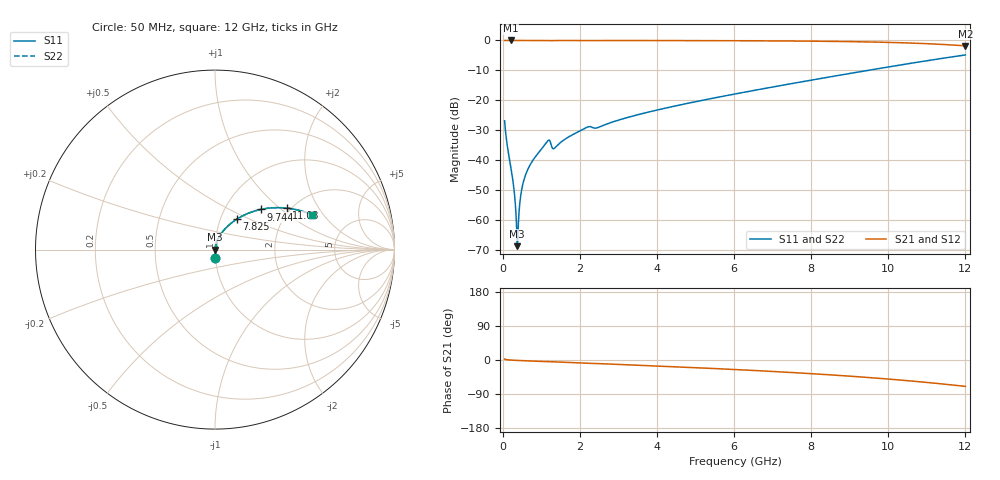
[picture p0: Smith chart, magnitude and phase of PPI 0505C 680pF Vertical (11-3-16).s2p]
# GHz S MA R 50
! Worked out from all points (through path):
!   1601 points, 50 MHz to 12 GHz, reference 50 ohm
!   highest |S21| = 0.00 dB at 214.3 MHz (marker M1); lowest = -1.8 dB at 12 GHz (marker M2)
!   group delay of S21, straight-line fit = 15.2 ps
!   lowest |S11| = -68.6 dB at 378.6 MHz (marker M3), VSWR 1.00, Z = 50 - j0.00888 ohm
!   |S11| at or under -10 dB: start of sweep to 9.462 GHz
!   |S22| runs from -68.6 to -4.8 dB; largest |S21 - S12| = 0
!   S11 on the Smith chart (normalised r, x): 50 MHz: 1.00, -0.09; 7.825 GHz: 1.19, +0.42; 9.744 GHz: 1.46, +0.74; 11.03 GHz: 1.90, +1.12; 12 GHz: 2.68, +1.56
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0.05  0.04591 -87.3  0.9987 2.5  0.9987 2.5  0.04591 -87.3
0.2143125  0.007481 -87.9  0.9997 -0.2  0.9997 -0.2  0.007481 -87.9
0.2815313  0.003802 -85.7  0.9996 -0.6  0.9996 -0.6  0.003802 -85.7
0.3412812  0.00141 -76.6  0.9996 -0.9  0.9996 -0.9  0.00141 -76.6
0.378625  0.0003727 -13.8  0.9996 -1.1  0.9996 -1.1  0.0003727 -13.8
0.4159687  0.001147 69.5  0.9996 -1.3  0.9996 -1.3  0.001147 69.5
0.4831875  0.003002 80.7  0.9996 -1.6  0.9996 -1.6  0.003002 80.7
0.5504062  0.004708 82.9  0.9995 -1.9  0.9995 -1.9  0.004708 82.9
0.6624375  0.00734 84.0  0.9995 -2.4  0.9995 -2.4  0.00734 84.0
0.8192812  0.01086 84.0  0.9993 -3.1  0.9993 -3.1  0.01086 84.0
1.162844  0.02094 74.3  0.9957 -4.6  0.9957 -4.6  0.02094 74.3
1.342094  0.01596 71.5  0.996 -4.9  0.996 -4.9  0.01596 71.5
2.044156  0.03209 79.1  0.9977 -7.9  0.9977 -7.9  0.03209 79.1
2.454938  0.03506 74.4  0.9954 -9.3  0.9954 -9.3  0.03506 74.4
4.038312  0.07005 73.0  0.996 -16.0  0.996 -16.0  0.07005 73.0
6.025  0.1282 64.2  0.9898 -25.1  0.9898 -25.1  0.1282 64.2
7.824969  0.2082 54.5  0.9755 -35.0  0.9755 -35.0  0.2082 54.5
8.019156  0.219 53.3  0.973 -36.1  0.973 -36.1  0.219 53.3
9.744438  0.3392 41.3  0.9369 -48.2  0.9369 -48.2  0.3392 41.3
10.01331  0.3625 39.1  0.928 -50.4  0.928 -50.4  0.3625 39.1
11.02906  0.4621 30.0  0.8818 -59.5  0.8818 -59.5  0.4621 30.0
12  0.5736 19.8  0.8128 -69.6  0.8128 -69.6  0.5736 19.8
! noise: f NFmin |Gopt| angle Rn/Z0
0.05  0.0003131  0.8343  0.1924  0.000399
1.372  0.006342  0.782  4.056  0.005961
2.701  0.007019  0.643  7.797  0.003703
4.031  0.007369  0.5294  11.1  0.002734
5.36  0.009191  0.5078  14.37  0.003196
6.682  0.01135  0.5067  17.51  0.003907
8.012  0.01398  0.5199  20.59  0.004947
9.341  0.01733  0.546  23.69  0.006534
10.67  0.02188  0.585  26.88  0.009138
12  0.02854  0.6371  30.28  0.01386
